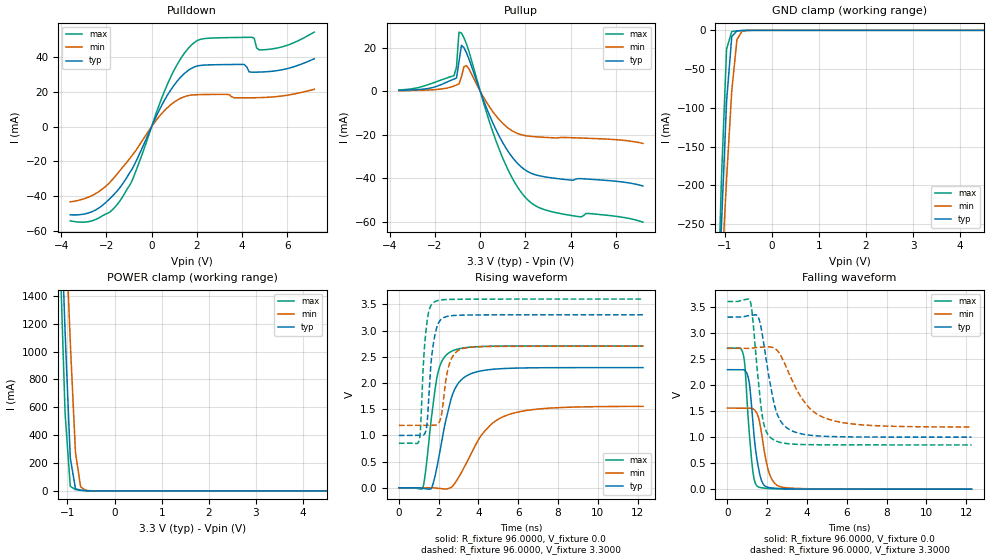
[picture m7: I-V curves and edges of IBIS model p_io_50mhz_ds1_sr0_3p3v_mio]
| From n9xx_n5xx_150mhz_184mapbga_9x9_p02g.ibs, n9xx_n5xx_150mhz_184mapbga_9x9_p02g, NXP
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[Model] p_io_50mhz_ds1_sr0_3p3v_mio
|   Model p_io_50mhz_ds1_sr0_3p3v_mio
| This model was characterised for following simulation conditions:
| External (pad) voltage:
|   - Typ: 3.3V,   - Min: 2.7V,   - Max: 3.6V
| Library cells for typ/min/max conditions are connected as defined below:
|  pad - External Pad
|  ipp_do_lv - Core Input
|  ipp_obe_lv - Output Buffer Enable
|  IOGC - NC
|  REFH3V3 - REFH3V3
|  REFL3V3 - REFL3V3
|  ZI - NC
|  abut_ncal_vddio[1] - vddio
|  abut_ncal_vddio[2] - vddio
|  abut_ncal_vddio[3] - vssio
|  abut_ncal_vddio[4] - vddio
|  abut_ncal_vddio[5] - vddio
|  abut_ncal_vddio[6] - vssio
|  abut_pcal_vddio[1] - vssio
|  abut_pcal_vddio[2] - vssio
|  abut_pcal_vddio[3] - vddio
|  abut_pcal_vddio[4] - vssio
|  abut_pcal_vddio[5] - vssio
|  abut_pcal_vddio[6] - vddio
|  ipp_do_1p8v - ipp_do_1p8v
|  ipp_dse_lv - vdd_lv
|  ipp_eftd_lv - NC
|  ipp_ina_mux_vddio - NC
|  ipp_ina_mux_vddio[0] - NC
|  ipp_ina_mux_vddio[1] - NC
|  ipp_ina_r0_vddio - NC
|  ipp_ina_r0a_vddio - NC
|  ipp_ina_r0b_vddio - NC
|  ipp_ina_r0c_vddio - NC
|  ipp_ina_r0d_vddio - NC
|  ipp_ina_r0e_vddio - NC
|  ipp_ina_r0f_vddio - NC
|  ipp_ina_r300_vddio - NC
|  ipp_ina_r300a_vddio - NC
|  ipp_ina_r300b_vddio - NC
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Model_type I/O
Polarity   Non-Inverting
Enable   Active-High
Vinl =   0.9900V
Vinh =   2.3100V
Vmeas =  1.6500V
Cref =   30.0000pF
Rref =   1.0000M
Vref =   3.3000V
C_comp   1.4363pF   1.3758pF   1.5227pF
|C_comp_pullup   0.7200pF   0.7523pF   0.6981pF
|C_comp_pulldown   0.6275pF   0.6820pF   0.5882pF
[Model Spec]
| variable   typ   min   max
Vinh   2.3100V   1.8900V   2.5200V
Vinl   0.9900V   0.8100V   1.0800V
[Temperature Range]   25.0000   0.1250k   -40.0000
[Voltage Range]   3.3000V   2.7000V   3.6000V
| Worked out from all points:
|   slope of the pulldown table from 0 to 0.495 V, typ, clamps not added: 36.8 ohm
|   slope of the pullup table from 0 to 0.495 V, typ, clamps not added: 37.8 ohm
|   GND clamp passes 1 mA (typ) near -0.74 V on its own axis
|   POWER clamp passes 1 mA (typ) near -0.54 V on its own axis
|   rising waveform, R_fixture 96.0000, V_fixture 0.0: 20-80 % time 804ps typ, 1.57ns min, 530ps max; typ from 0 V to 2.29 V
|   rising waveform, R_fixture 96.0000, V_fixture 3.3000: 20-80 % time 313ps typ, 388ps min, 255ps max; typ from 0.998 V to 3.3 V
|   falling waveform, R_fixture 96.0000, V_fixture 0.0: 20-80 % time 375ps typ, 456ps min, 303ps max; typ from 2.29 V to 0 V
|   falling waveform, R_fixture 96.0000, V_fixture 3.3000: 20-80 % time 677ps typ, 1.41ns min, 428ps max; typ from 3.3 V to 0.998 V
[Pulldown]
|Voltage   I(typ)   I(min)   I(max)
-3.6V     -50.71mA   -43.27mA   -54.18mA
-2.5V     -48.1mA    -38.69mA   -53.56mA
-1.4V     -35.02mA   -25.26mA   -42.7mA
-850mV    -24.18mA   -16.32mA   -30.7mA
800mV     20.23mA    12.14mA    27.32mA
1.9V      34.45mA    18.38mA    48.57mA
4.1V      35.83mA    16.63mA    51.44mA
4.43V     31.42mA    16.66mA    51.52mA
4.54V     31.41mA    16.69mA    50.94mA
4.65V     31.42mA    16.71mA    45.28mA
5.09V     31.67mA    16.92mA    44.44mA
7.2V      39.12mA    21.58mA    54.49mA
[Pullup]
|Voltage   I(typ)   I(min)   I(max)
-3.6V     390.2uA    234.7uA    600.5uA
-1.16V    5.607mA    2.418mA    7.152mA
-1.05V    6.059mA    2.87mA     11.01mA
-940mV    13.57mA    3.339mA    27.22mA
-830mV    21.13mA    6.682mA    26.77mA
-720mV    20.02mA    11.25mA    24.57mA
-610mV    17.72mA    11.8mA     21.82mA
820mV     -20.27mA   -12.85mA   -26.19mA
1.48V     -31.2mA    -18.62mA   -41.17mA
2.03V     -36.53mA   -20.52mA   -49.25mA
3.46V     -40.29mA   -21.45mA   -56.15mA
7.2V      -43.65mA   -24.03mA   -60.31mA
[GND_clamp]
|Voltage   I(typ)   I(min)   I(max)
-3.6V     -4.967A    -3.834A    -6.451A
-1.18V    -432.4mA   -454.2mA   -428.7mA
-1.07V    -252.8mA   -319.9mA   -193.4mA
-960mV    -91.54mA   -192mA     -24.27mA
-850mV    -8.013mA   -77.89mA   -1.462mA
-740mV    -731.9uA   -11.92mA   -724.8uA
-630mV    -284.5uA   -928.5uA   -315.1uA
-300mV    -508.9nA   -3.038uA   -108.6nA
7.2V      0A         0A         0A
[POWER_clamp]
|Voltage   I(typ)   I(min)   I(max)
-3.6V     26.34A     23.98A     28.82A
-1.16V    2.208A     2.937A     1.722A
-1.05V    1.14A      1.999A     556.4mA
-940mV    237.9mA    1.069A     33.46mA
-830mV    16.33mA    277.1mA    9.216mA
-720mV    4.663mA    29.2mA     4.86mA
-610mV    1.877mA    3.923mA    1.821mA
7.2V      0A         0A         0A
[Ramp]
| variable   typ   min   max
dV/dt_r  1.3753/0.8045n   0.9320/1.5748n   1.6230/0.5304n
dV/dt_f  1.3810/0.6775n   0.9049/1.4130n   1.6509/0.4278n
R_load = 96.0000
[Rising Waveform]
R_fixture= 96.0000
V_fixture= 0.0
V_fixture_min= 0.0
V_fixture_max= 0.0
|time   V(typ)   V(min)   V(max)
0s        4.193nV    211.1nV    14.22nV
1.201ns   -9.215mV   -138.7uV   -7.749mV
1.36ns    -19mV      275.2uV    361mV
1.64ns    -7.055mV   400.2uV    1.348V
1.942ns   444.5mV    -9.588mV   2.158V
2.599ns   1.66V      1.18mV     2.594V
3.366ns   2.126V     449.2mV    2.674V
4.208ns   2.235V     1.033V     2.696V
5.345ns   2.276V     1.372V     2.703V
12.27ns   2.292V     1.553V     2.705V
[Rising Waveform]
R_fixture= 96.0000
V_fixture= 3.3000
V_fixture_min= 2.7000
V_fixture_max= 3.6000
|time   V(typ)   V(min)   V(max)
0s        998.1mV    1.19V      848.4mV
1.025ns   999.9mV    1.19V      910.3mV
1.251ns   1.008V     1.19V      2.483V
1.369ns   1.104V     1.191V     3.015V
1.618ns   2.387V     1.191V     3.481V
1.796ns   2.882V     1.19V      3.547V
2.121ns   3.212V     1.348V     3.583V
2.553ns   3.278V     2.377V     3.594V
3.104ns   3.293V     2.643V     3.597V
12.27ns   3.3V       2.7V       3.6V
[Falling Waveform]
R_fixture= 96.0000
V_fixture= 0.0
V_fixture_min= 0.0
V_fixture_max= 0.0
|time   V(typ)   V(min)   V(max)
0s        2.292V     1.555V     2.705V
805.1ps   2.291V     1.555V     2.566V
891.8ps   2.272V     1.555V     2.289V
1.071ns   2.095V     1.556V     1.194V
1.245ns   1.411V     1.549V     436.8mV
1.538ns   447.6mV    1.398V     46.83mV
1.762ns   121.2mV    945.1mV    23.22mV
2.071ns   31.33mV    337.9mV    12.37mV
2.638ns   11.69mV    47.32mV    4.457mV
12.27ns   36.74uV    74.81uV    26.09uV
[Falling Waveform]
R_fixture= 96.0000
V_fixture= 3.3000
V_fixture_min= 2.7000
V_fixture_max= 3.6000
|time   V(typ)   V(min)   V(max)
0s        3.3V       2.7V       3.6V
1.14ns    3.332V     2.701V     3.613V
1.266ns   3.337V     2.707V     3.287V
1.523ns   3.317V     2.719V     2.184V
1.748ns   2.975V     2.725V     1.408V
2.299ns   1.72V      2.715V     950.6mV
3.007ns   1.169V     2.297V     873.4mV
3.946ns   1.045V     1.632V     854.2mV
4.872ns   1.014V     1.369V     850.3mV
12.27ns   998.3mV    1.192V     848.5mV
